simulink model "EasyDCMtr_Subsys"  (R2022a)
settings: Solver=VariableStepAuto  StartTime=0.0  StopTime=10.0  RelTol=1e-3
libraries: simulink x1

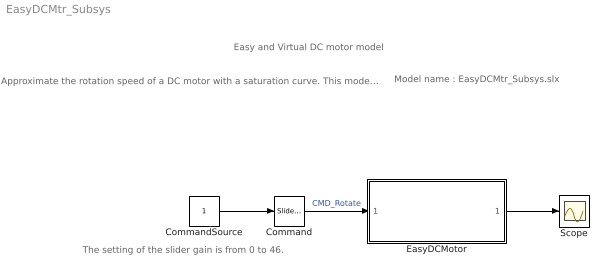
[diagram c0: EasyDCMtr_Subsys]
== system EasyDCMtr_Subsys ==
  note: The setting of the slider gain is from 0 to 46.
  note: Approximate the rotation speed of a DC motor with a saturation curve. This model specifies a rotation speed command (0 to 46rad/s) with a slider gain.
  note: Model name : EasyDCMtr_Subsys.slx
  note: Easy and Virtual DC motor model
  Command : simulink/Math Operations/Slider Gain  gain=46.0  low=0  high=46
  CommandSource : Constant
  EasyDCMotor : Subsystem
  Scope : Scope
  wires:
  CommandSource/1 -> Command/1
  Command/1 -> EasyDCMotor/1(CMD_Rotate)  "CMD_Rotate"
  EasyDCMotor/1(Rotate) -> Scope/1

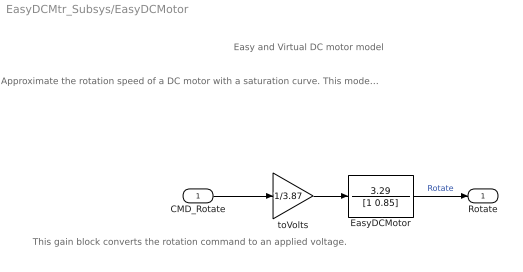
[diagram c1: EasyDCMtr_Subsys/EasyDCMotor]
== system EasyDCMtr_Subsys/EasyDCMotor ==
  note: This gain block converts the rotation command to an applied voltage.
  note: Approximate the rotation speed of a DC motor with a saturation curve. This model is not an exact mathematical model.
  note: Easy and Virtual DC motor model
  CMD_Rotate : Inport
  EasyDCMotor : TransferFcn  Numerator=3.29  Denominator=[1 0.85]
  toVolts : Gain  Gain=1/3.87
  Rotate : Outport
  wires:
  toVolts/1 -> EasyDCMotor/1
  CMD_Rotate/1 -> toVolts/1
  EasyDCMotor/1 -> Rotate/1  "Rotate"
